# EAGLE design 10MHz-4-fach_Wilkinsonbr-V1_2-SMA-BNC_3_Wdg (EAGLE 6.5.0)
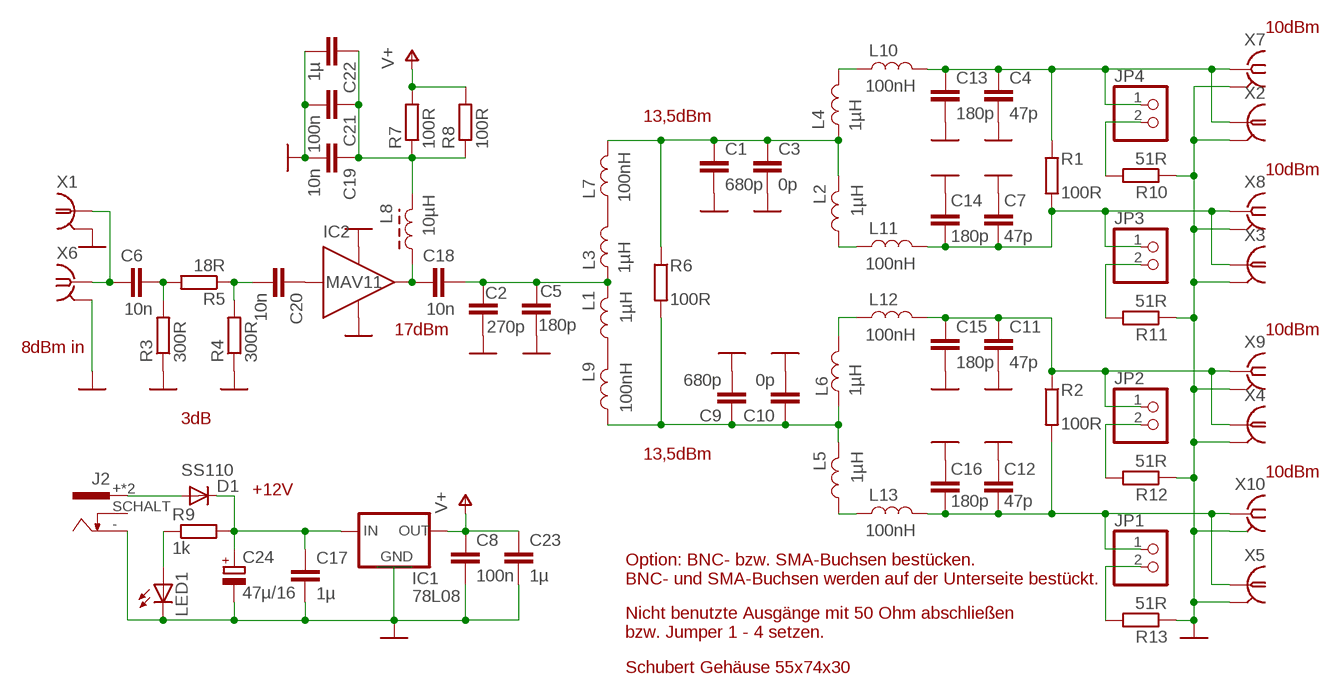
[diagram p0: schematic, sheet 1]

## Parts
C1  680p  C-EUC1206  [C1206]
C2  270p  C-EUC1206  [C1206]
C3  0p  C-EUC1206  [C1206]
C4  47p  C-EUC1206  [C1206]
C5  180p  C-EUC1206  [C1206]
C6  10n  C-EUC1206  [C1206]
C7  47p  C-EUC1206  [C1206]
C8  100n  C-EUC1206  [C1206]
C9  680p  C-EUC1206  [C1206]
C10  0p  C-EUC1206  [C1206]
C11  47p  C-EUC1206  [C1206]
C12  47p  C-EUC1206  [C1206]
C13  180p  C-EUC1206  [C1206]
C14  180p  C-EUC1206  [C1206]
C15  180p  C-EUC1206  [C1206]
C16  180p  C-EUC1206  [C1206]
C17  1µ  C-EUC1206  [C1206]
C18  10n  C-EUC1206  [C1206]
C19  10n  C-EUC1206  [C1206]
C20  10n  C-EUC1206  [C1206]
C21  100n  C-EUC1206  [C1206]
C22  1µ  C-EUC1206  [C1206]
C23  1µ  C-EUC1206  [C1206]
C24  47µ/16  CPOL-EUC/6032-28R  [C/6032-28R]
D1  SS110  DIODE-MELF-MLL41  [MELF-MLL41]
IC1  78L08  78XXLOB  [SO-08]
IC2  MAV11  MAV1  [MAV]
J2  HOHLBUCHSE-SMT-INVERS  [HOHLBUCHSESMT+INNEN]
JP1  PINHD-1X2  [1X02]
JP2  PINHD-1X2  [1X02]
JP3  PINHD-1X2  [1X02]
JP4  PINHD-1X2  [1X02]
L1  1µH  L-3_WDG  [L3230M]
L2  1µH  L-3_WDG  [L3230M]
L3  1µH  L-3_WDG  [L3230M]
L4  1µH  L-3_WDG  [L3230M]
L5  1µH  L-3_WDG  [L3230M]
L6  1µH  L-3_WDG  [L3230M]
L7  100nH  L-3_WDG  [L3230M]
L8  10µH  L-3-WDG-FERRIT  [L3230M]
L9  100nH  L-3_WDG  [L3230M]
L10  100nH  L-3_WDG  [L3230M]
L11  100nH  L-3_WDG  [L3230M]
L12  100nH  L-3_WDG  [L3230M]
L13  100nH  L-3_WDG  [L3230M]
LED1  NFSG036BT  [NFSG036BT]
R1  100R  R-EU_R1206  [R1206]
R2  100R  R-EU_R1206  [R1206]
R3  300R  R-EU_R1206  [R1206]
R4  300R  R-EU_R1206  [R1206]
R5  18R  R-EU_R1206  [R1206]
R6  100R  R-EU_R1206  [R1206]
R7  100R  R-EU_R1206  [R1206]
R8  100R  R-EU_R1206  [R1206]
R9  1k  R-EU_R1206  [R1206]
R10  51R  R-EU_R1206  [R1206]
R11  51R  R-EU_R1206  [R1206]
R12  51R  R-EU_R1206  [R1206]
R13  51R  R-EU_R1206  [R1206]
X1  1-227161-0  [AMP_227161]
X2  1-227161-0  [AMP_227161]
X3  1-227161-0  [AMP_227161]
X4  1-227161-0  [AMP_227161]
X5  1-227161-0  [AMP_227161]
X6  BU-SMA-H  [BU-SMA-H]
X7  BU-SMA-H  [BU-SMA-H]
X8  BU-SMA-H  [BU-SMA-H]
X9  BU-SMA-H  [BU-SMA-H]
X10  BU-SMA-H  [BU-SMA-H]

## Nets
GND: C1.2 C2.2 C3.2 C4.2 C5.2 C7.2 C8.2 C9.2 C10.2 C11.2 C12.2 C13.2 C14.2 C15.2 C16.2 C17.2 C19.2 C21.2 C22.2 C23.2 C24.- IC1.2(GND) IC1.3(GND) IC1.6(GND) IC1.7(GND) IC2.GND1 IC2.GND2 J2.-(+) LED1.C R3.1 R4.1 R10.1 R11.1 R12.1 R13.1 X1.2 X2.2 X3.2 X4.2 X5.2 X7.2 X7.3 X7.4 X7.5 X8.2 X8.3 X8.4 X8.5 X9.2 X9.3 X9.4 X9.5 X10.2 X10.3 X10.4 X10.5
N$1: C1.1 C3.1 L2.2 L4.1 L7.2 R6.1
N$2: C7.1 C14.1 JP3.1 L11.2 R1.2 X3.1 X8.1
N$3: C2.1 C5.1 C18.2 L1.2 L3.1
N$4: C4.1 C13.1 JP4.1 L10.2 R1.1 X2.1 X7.1
N$5: C9.1 C10.1 L5.2 L6.1 L9.1 R6.2
N$6: C12.1 C16.1 JP1.1 L13.2 R2.2 X5.1 X10.1
N$7: C11.1 C15.1 JP2.1 L12.2 R2.1 X4.1 X9.1
N$8: C20.2 R4.2 R5.1
N$9: C6.2 R3.2 R5.2
N$10: C6.1 X1.1 X6.1
N$11: L3.2 L7.1
N$12: LED1.A R9.1
N$13: C17.1 C24.+ D1.C IC1.8(IN) R9.2
N$14: L1.1 L9.2
N$15: L4.2 L10.1
N$16: C20.1 IC2.IN
N$17: C19.1 C21.1 C22.1 L8.2 R7.1 R8.1
N$18: C18.1 IC2.OUT L8.1
N$19: L6.2 L12.1
N$20: L5.1 L13.1
N$21: L2.1 L11.1
N$22: JP4.2 R10.2
N$23: JP3.2 R11.2
N$24: JP2.2 R12.2
N$25: JP1.2 R13.2
N$26: D1.A J2.+(-) J2.@+(-)
V+: C8.1 C23.1 IC1.1(OUT) R7.2 R8.2
Unconnected: J2.SCHALT X6.2 X6.3 X6.4 X6.5

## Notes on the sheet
- 10dBm
- 13,5dBm
- 10dBm
- 17dBm | 10dBm
- 8dBm in
- 3dB
- 13,5dBm
- 10dBm
- +12V
- Option: BNC- bzw. SMA-Buchsen bestücken.
  BNC- und SMA-Buchsen werden auf der Unterseite bestückt.
- Nicht benutzte Ausgänge mit 50 Ohm abschließen
  bzw. Jumper 1 - 4 setzen.
- Schubert Gehäuse 55x74x30

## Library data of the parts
C1-C23 = rcl:C-EU: CAPACITOR, European symbol
C24 = rcl:CPOL-EU: POLARIZED CAPACITOR, European symbol
D1 = diode:DIODE-: DIODE
IC1 = dk3ha-2015-01:78XXLOB: Gehäuse SO-08
IC2 = dk3ha-2015-01:MAV1
J2 = dk3ha-2015-01:HOHLBUCHSE-SMT-INVERS: Innenstift Minuspol
JP1-JP4 = pinhead:PINHD-1X2: PIN HEADER
L1-L7 L9-L13 = rcl:L-3_WDG
L8 = rcl:L-3-WDG-FERRIT
LED1 = led:NFSG036BT: CHIP TYPE GREEN LED NFSx036xT
R1-R13 = rcl:R-EU_: RESISTOR, European symbol
X1-X5 = con-coax:?227161*: JACK, RIGHT ANGLE, 50 OHM, PCB, BNC; MF: TYCO ELECTRONICS; MPN: 1-227161; OC_FARNELL: unknown; OC_NEWARK: 33B3200
X6-X10 = con-coax:BU-SMA-H: FEMALE SMA CONNECTOR; OC_FARNELL: unknown; OC_NEWARK: unknown

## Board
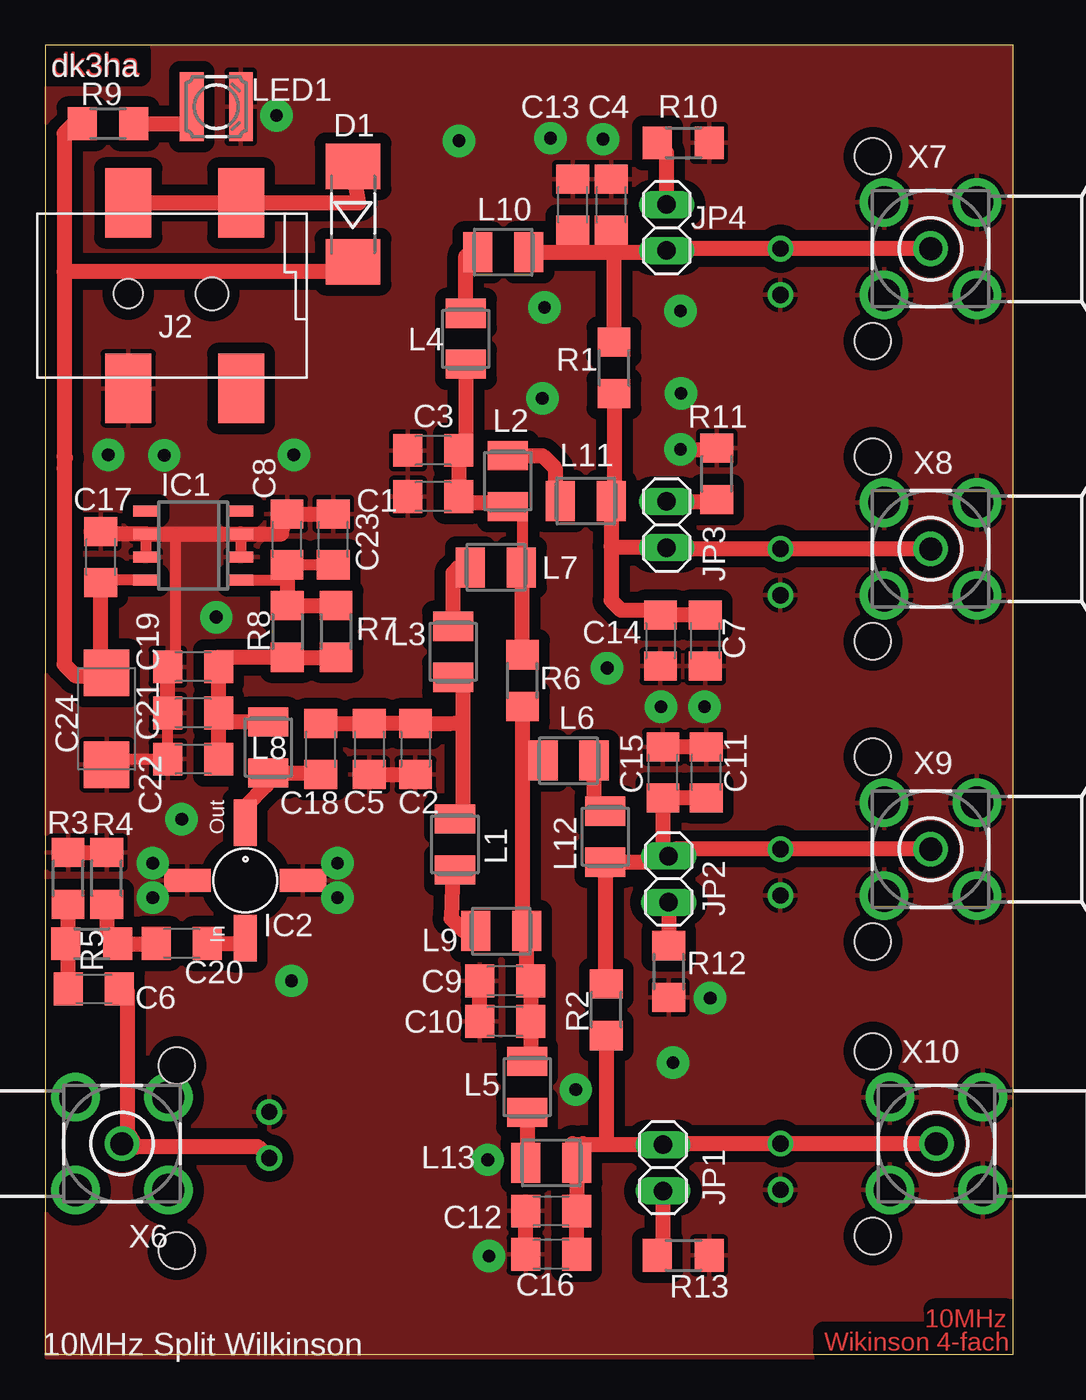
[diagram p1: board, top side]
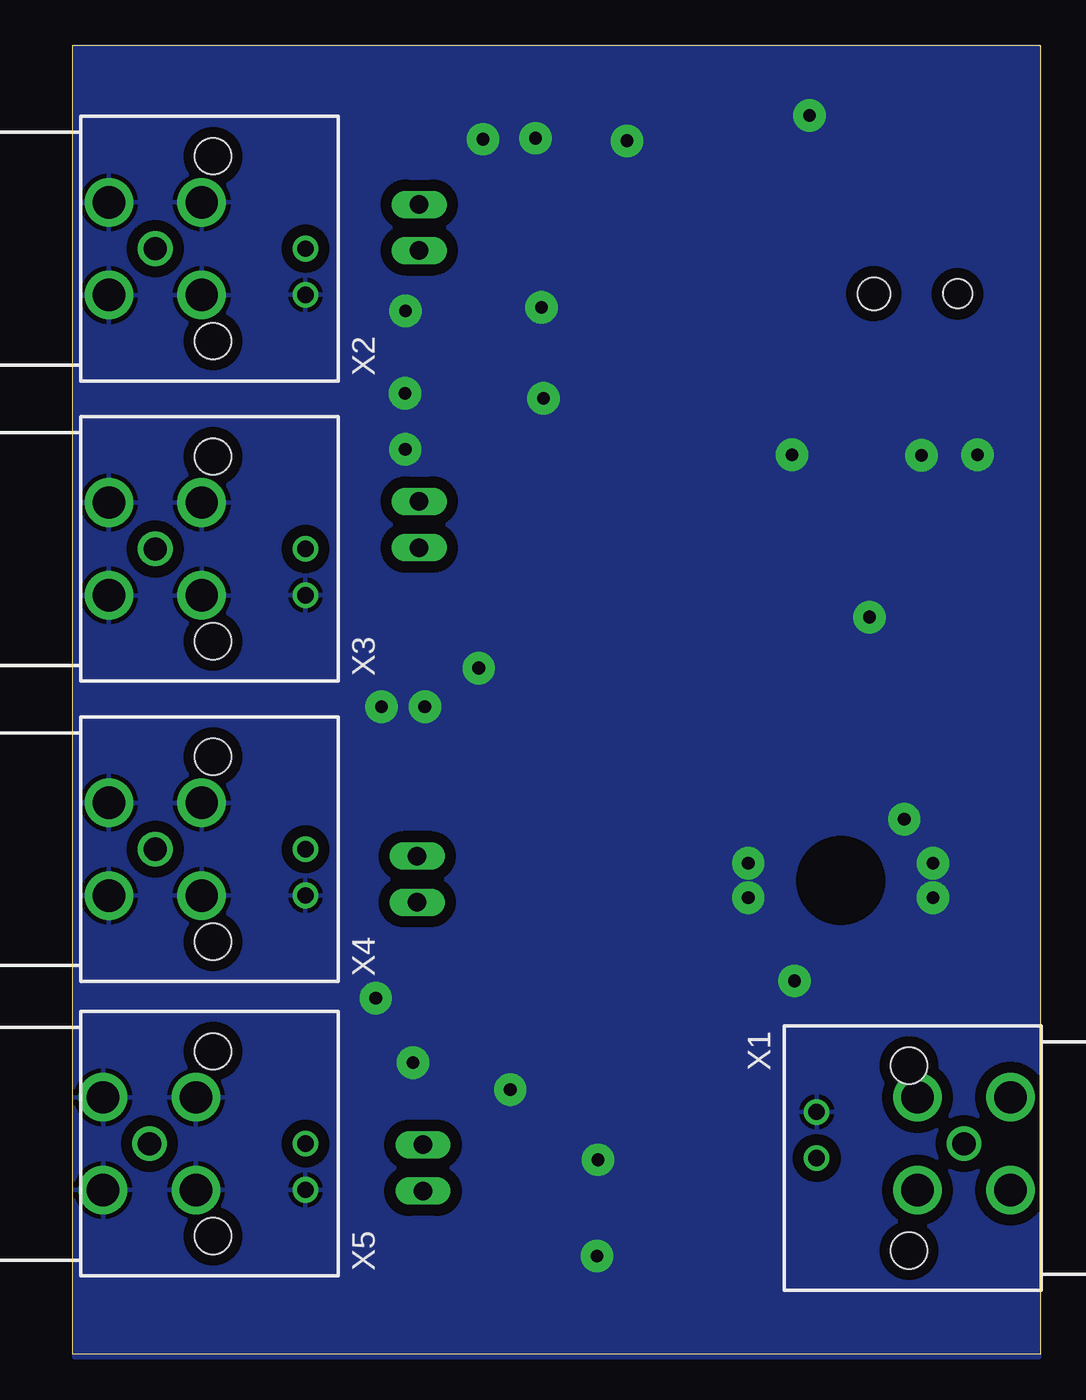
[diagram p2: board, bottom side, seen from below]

Size 53.19 x 71.95 mm. Coordinates in mm from the lower left corner, seen from the top.
Outline: 0,0 53.19,0 53.19,71.95 0,71.95 0,0
Copper layers (1*16): Top 0.035mm / dielectric 1.5mm / Bottom 0.035mm
Design rules "default *": minimum track width 10mil, minimum drill 24mil, track to track 8mil, track to pad 8mil, pad to pad 8mil, via to via 8mil, smd to smd 8mil, copper to edge 0mil, drill to drill 8mil, minimum pad ring 10mil, minimum via ring 8mil, stop-mask expansion 4mil, vias tented up to drill 0mil, thermal gap 10mil

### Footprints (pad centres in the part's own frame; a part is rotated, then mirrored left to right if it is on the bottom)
C1206 = smd 1.6 x 1.8: 1 -1.4,0; 2 1.4,0
C/6032-28R = smd 2.55 x 2.5: + 2.525,0; - -2.525,0
MELF-MLL41 = smd 2.5 x 3: A 2.625,0; C -2.625,0
SO-08 = smd 0.6 x 1.4: 1 -1.905,-2.6; 2 -0.635,-2.6; 3 0.635,-2.6; 4 1.905,-2.6; 5 1.905,2.6; 6 0.635,2.6; 7 -0.635,2.6; 8 -1.905,2.6
MAV = smd 1.27 x 2.54: GND1 0,3.175; GND2 0,-3.175 | smd 2.54 x 1.27: IN -3.175,0; OUT 3.175,0
HOHLBUCHSESMT+INNEN = smd 2.54 x 3.81: + 1.19,4.52; - 1.19,-5.68; @+ 7.39,4.52; SCHALT 7.39,-5.68 | hole 1.6: 1.19,-0.48 | hole 1.8: 5.79,-0.48
1X02 = drill 1.016 long: 1 -1.27,0; 2 1.27,0
L3230M = smd 1.6 x 2.2: 1 -1.4,0; 2 1.4,0
NFSG036BT = smd 1.3 x 3.8: A 1.35,0; C -1.35,0
R1206 = smd 1.6 x 1.803: 1 -1.422,0; 2 1.422,0
AMP_227161 = drill 0.9 pad 1.27: 1 0,-5.08; 2 -2.54,-5.08 | hole 2: -5.08,0; 5.08,0
BU-SMA-H = drill 1.27: 1 0,0 | drill 1.778: 2 -2.55,2.55; 3 2.55,2.55; 4 2.55,-2.55; 5 -2.55,-2.55

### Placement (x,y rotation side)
C1  21.32,47.15 180 top
C2  20.34,33.27 270 top
C3  21.32,49.69 180 top
C4  31.1,63.2 90 top
C5  17.8,33.27 270 top
C6  2.66,20.07 180 top
C7  36.26,39.23 270 top
C8  13.28,44.8 90 top
C9  25.27,20.52 180 top
C10  25.27,18.3 180 top
C11  36.32,31.99 90 top
C12  27.8,7.87 180 top
C13  28.98,63.2 90 top
C14  33.8,39.23 270 top
C15  33.94,31.99 90 top
C16  27.8,5.48 180 top
C17  3.04,43.82 90 top
C18  15.13,33.27 90 top
C19  8.12,37.79 180 top
C20  7.49,22.58 180 top
C21  8.12,35.25 180 top
C22  8.12,32.71 180 top
C23  15.82,44.8 90 top
C24  3.36,34.93 90 top
D1  16.9,62.69 90 top
IC1  8.12,44.46 90 top
IC2  10.98,26.04 90 top
J2  3.36,58.78 0 top
JP1  33.94,10.24 270 top
JP2  34.26,26.11 270 top
JP3  34.15,45.61 90 top
JP4  34.15,61.94 90 top
L1  22.51,28.02 90 top
L2  25.41,48 270 top
L3  22.41,38.62 90 top
L4  23.1,55.82 90 top
L5  26.48,14.68 90 top
L6  28.75,32.63 0 top
L7  24.76,43.26 0 top
L8  12.25,33.34 90 top
L9  25.05,23.26 180 top
L10  25.17,60.59 0 top
L11  29.69,46.9 0 top
L12  30.77,28.45 270 top
L13  27.8,10.52 0 top
LED1  9.39,68.59 180 top
R1  31.26,54.23 270 top
R2  30.82,18.93 270 top
R3  1.24,26.15 270 top
R4  3.36,26.15 270 top
R5  2.54,22.56 180 top
R6  26.22,37.03 270 top
R7  15.97,39.73 90 top
R8  13.3,39.73 90 top
R9  3.44,67.66 180 top
R10  35.05,66.6 180 top
R11  36.9,48.4 270 top
R12  34.26,21.03 90 top
R13  35.06,5.43 180 top
X1  7.22,10.77 270 bottom
X2  45.48,60.78 90 bottom
X3  45.48,44.27 90 bottom
X4  45.48,27.76 90 bottom
X5  45.48,11.57 90 bottom
X6  4.2,11.57 180 top
X7  48.65,60.78 0 top
X8  48.65,44.27 0 top
X9  48.65,27.76 0 top
X10  48.97,11.57 0 top

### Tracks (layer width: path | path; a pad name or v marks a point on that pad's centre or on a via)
GND  (via drill 0.7 pad 1.78)
  Top 0.61: IC1.6 IC1.7 | IC1.3 IC1.2 | C19.2 7.17,38.11 7.17,45.09 | 3.17,45.09 C17.2 | C21.2 C22.2 3.36,32.71 3.04,32.39 C24.-
  Top 0.813: C5.2 C2.2 | C10.2 C9.2 | C16.2 C12.2 | 3.17,45.09 IC1.6 7.17,45.09 IC1.3 12.96,45.09 C8.2 C23.2 | C21.2 C19.2 | R3.1 R4.1 | C11.2 C15.2 | v34.91,49.74 36.81,49.74 R11.1
  other vias: 5.9,25.09 16.06,27 22.73,66.71 27.31,52.55 13.52,20.52 24.37,5.38 30.64,66.8 24.31,10.68 27.43,57.55 34.91,57.36 16.06,25.09 5.9,27 12.7,68.1 36.22,35.6 34.49,16.03 30.87,37.72 3.45,49.44 6.53,49.41 13.65,49.44 29.15,14.55 36.54,19.56 34.93,52.82 33.84,35.6 27.76,66.86 9.39,40.52 7.48,29.41
  pour Top (isolate 0.61): 0.07,71.89 53.1,71.89 53.1,-0.18 0.07,-0.18
  pour Bottom (isolate 0.61): 0.07,71.89 53.1,71.89 53.1,-0.18 0.07,-0.18
N$1
  Top 0.406: L2.2 26.23,46.6 26.23,46.51
  Top 0.61: L7.2 26.3,43.26 26.3,42.96 | 26.38,43.38 26.23,43.38 26.23,46.51
  Top 0.813: R6.1 26.22,42.59 26.3,42.96 26.38,43.38 | 22.47,46.76 C1.1 | C1.1 C3.1 23.1,50.07 L4.1 | C1.1 22.94,47.15 22.94,46.81 25.41,46.81 L2.2
N$2
  Top 0.813: C7.1 C14.1 33.52,40.91 31.63,40.91 31.09,41.44 31.09,44.41 | 34.6,44.38 JP3.1 | 31.09,44.41 L11.2 31.26,47.06 R1.2 | JP3.1 31.16,44.34 31.09,44.41 | 34.15,44.27 JP3.1 | X8.1 X3.1 34.21,44.27 JP3.1
N$3
  Top 0.813: C18.2 C5.1 C2.1 22.22,34.66 22.94,34.75 | 22.94,34.75 22.94,37.29 22.23,37.22 L3.1 | 22.94,34.75 22.94,29.43 22.51,29.75 L1.2
N$4
  Top 0.254: 28.98,60.6 28.97,60.59 | 31.1,60.61 31.13,60.59
  Top 0.813: L10.2 28.97,60.59 31.13,60.59 | 31.13,60.59 34.06,60.59 JP4.1 | 34.3,60.82 JP4.1 | R1.1 31.26,60.46 31.13,60.59 | C13.1 28.98,60.6 | C4.1 31.1,60.61 | 34.15,60.78 JP4.1 | X7.1 X2.1 34.25,60.78 JP4.1
N$5
  Top 0.813: R6.2 26.22,32.52 | 26.22,32.52 26.22,23.82 26.45,23.82 L9.1 26.45,20.52 C9.1 C10.1 26.66,16.07 26.49,16.07 L5.2 | L6.1 26.33,32.63 26.22,32.52
N$6
  Top 0.813: C16.1 C12.1 L13.2 28.97,10.75 28.97,11.57 29.03,11.51 29.6,11.51 | JP1.1 30.87,11.51 | 30.87,11.51 29.6,11.51 | 29.55,11.56 29.6,11.51 | R2.2 30.82,11.56 30.87,11.51 | 33.94,11.57 JP1.1 | X10.1 X5.1 34,11.57 JP1.1
N$7
  Top 0.813: JP2.1 33.92,27.05 L12.2 30.77,20.4 R2.1 | JP2.1 33.94,27.7 C15.1 C11.1 | 34.08,27.79 34.05,27.76 34.05,27.59 JP2.1 | 34.26,27.76 JP2.1 | X9.1 X4.1 34.63,27.76 JP2.1
N$8
  Top 0.813: R4.2 3.36,23.17 R5.1 6.08,22.56 C20.2
N$9
  Top 0.813: C6.2 1.26,22.68 | 1.26,22.68 1.26,24.71 R3.2 | R5.2 1.14,22.56 1.26,22.68
N$10
  Top 0.406: 5.02,11.39 4.2,11.39 4.2,11.41 X6.1
  Top 0.813: 5.02,11.39 4.52,12.2 4.52,19.93 C6.1 | 4.38,11.39 X6.1 | 4.2,11.41 11.66,11.41 X1.1
N$11
  Top 0.813: L3.2 22.4,42.87 22.4,42.95 22.78,43.32 L7.1
N$12
  Top 0.813: R9.1 8.02,67.66 LED1.A
N$13
  Top 0.406: 1.03,49.03 1.03,48.72
  Top 0.61: IC1.8 3.17,42.55 C17.1
  Top 0.813: C17.1 3.04,37.46 C24.+ 3.18,37.29 1.66,37.29 1.03,37.92 1.03,48.72 1.03,49.35 | R9.2 1.55,67.66 1.03,67.13 1.03,59.51 | 1.03,59.51 1.03,49.35 | 1.09,49.29 1.03,49.35 | D1.C 16.59,60.14 15.95,59.51 1.03,59.51
N$14
  Top 0.813: L1.1 22.38,26.62 22.3,23.95 22.99,23.26 L9.2
N$15
  Top 0.813: L4.2 23.1,60.37 L10.1
N$16
  Top 0.813: C20.1 10.69,22.58 IC2.IN
N$17
  Top 0.61: 9.28,37.68 9.21,37.68 9.71,37.66 | 9.97,34.75 C21.1
  Top 0.813: C22.1 C21.1 C19.1 | R7.1 R8.1 9.52,38.31 C19.1 | L8.2 9.97,34.75 | 9.71,37.66 9.52,37.66 C19.1
N$18
  Top 0.813: IC2.OUT 10.98,30.09 12.14,31.25 12.14,31.84 L8.1 15.37,31.95 C18.1
N$19
  Top 0.813: L6.2 30.15,30.47 L12.1
N$20
  Top 0.813: L5.1 26.48,10.59 L13.1
N$21
  Top 0.813: L2.1 27.33,49.4 28.02,48.72 28.02,47.18 L11.1
N$22
  Top 0.254: 34.15,66.09 R10.2
  Top 0.813: JP4.2 34.15,66.09
N$23
  Top 0.813: JP3.2 36.8,46.88 R11.2
N$24
  Top 0.813: JP2.2 R12.2
N$25
  Top 0.813: JP1.2 33.94,5.73 R13.2
N$26
  Top 0.813: J2.+ J2.@+ 17.22,63.3 D1.A
V+
  Top 0.61: C23.1 C8.1 | IC1.1 13.3,42.55
  Top 0.813: R7.2 R8.2 13.3,42.55 12.98,43.4 C8.1

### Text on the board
Top: dk3ha | 10MHz | Wikinson 4-fach
tPlace: dk3ha | 10MHz Split Wilkinson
